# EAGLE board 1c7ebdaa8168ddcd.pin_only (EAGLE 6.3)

Size 35.57 x 21.59 mm. Coordinates in mm from the lower left corner, seen from the top.
Outline: 0,19.05 0,2.54 arc90 2.54,0 33.02,0 arc90 35.56,2.54 35.56,19.05 arc90 33.4,21.59 2.54,21.59 arc90 0,19.05
Copper layers (1*16): Top 0.035mm / dielectric 1.5mm / Bottom 0.035mm
Design rules "adafruit *": minimum track width 8mil, minimum drill 15.5mil, track to track 8mil, track to pad 8mil, pad to pad 8mil, via to via 8mil, smd to smd 8mil, copper to edge 10mil, drill to drill 8mil, minimum pad ring 10mil, minimum via ring 8mil, stop-mask expansion 2mil, vias tented up to drill 20mil, thermal gap 10mil

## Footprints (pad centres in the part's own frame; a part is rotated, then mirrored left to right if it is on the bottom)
JSTPH2 = smd 1 x 4.6: 1 -1,-3.7; 2 1,-3.7 | smd 1.6 x 3.4: NC1 -3.4,1.5; NC2 3.4,1.5
0805-NO = smd 1.3 x 1.5: 1 -0.95,0; 2 0.95,0
EIA3528-21/B-R = smd 1.95 x 2.5: + 1.525,0; - -1.525,0
USB_HOST-PTH = drill 0.95 long: D+ 1,6.52; D- -1,6.52; GND 3.5,6.52; VBUS -3.5,6.52 | drill 2.3 pad 2.9: S1 -6.57,3.81; S2 6.57,3.81
FIDUCIAL_1MM = smd 1 x 1: 1 0,0
1X06-CLEANBIG = drill 1.016 pad 1.778 octagon: 1 -6.35,0; 2 -3.81,0; 3 -1.27,0; 4 1.27,0; 5 3.81,0; 6 6.35,0
1X02_ROUND = drill 1 pad 1.778: 1 -1.27,0; 2 1.27,0
INDUCTOR_5X5MM_TDK_VLC5045 = smd 2 x 5: P$1 -1.6,0; P$2 1.6,0
CHIPLED_0805_NOOUTLINE = smd 1.2 x 1.2: A 0,-1.05; C 0,1.05
SC59-BEC = smd 1 x 1.4: B -0.95,-1.2; C 0,1.2; E 0.95,-1.2
PVQFN-16 = smd 1.05 x 0.35: 1 -2.1,0.975; 2 -2.1,0.325; 3 -2.1,-0.325; 4 -2.1,-0.975; 9 2.1,-0.975; 10 2.1,-0.325; 11 2.1,0.325; 12 2.1,0.975 | smd 0.35 x 1.05: 5 -0.975,-2.1; 6 -0.325,-2.1; 7 0.325,-2.1; 8 0.975,-2.1; 13 0.975,2.1; 14 0.325,2.1; 15 -0.325,2.1; 16 -0.975,2.1 | drill 0.4: P$18 0,0; P$19 -0.9,0.9; P$20 0.9,0.9; P$21 0.9,-0.9; P$22 -0.9,-0.9 | smd 2.7 x 2.7: THERMAL 0,0
SOT23-5 = smd 0.55 x 1.2: 1 -0.95,-1.3; 2 0,-1.3; 3 0.95,-1.3; 4 0.95,1.3; 5 -0.95,1.3
MOUNTINGHOLE_2.5_PLATED = drill 2.5 pad 3.2: P$1 0,0
TERMBLOCK_1X2-3.5MM = drill 1 pad 2.184: 1 1.8,0; 2 -1.7,0
4UCONN_20329 = smd 1 x 2: BASE@1 -0.75,-2; BASE@2 0.75,-2 | smd 0.4 x 1.35: D+ 0,0.775; D- -0.65,0.775; GND 1.3,0.775; ID 0.65,0.775; VBUS -1.3,0.775 | drill 0.7 offset: SPRT@1 -3.3,0.9; SPRT@2 3.3,0.9 | drill 0.6 pad 2.5 square: SPRT@3 -3.6,-1.9; SPRT@4 3.6,-1.9 | hole 0.7: -1.95,0; 1.95,0

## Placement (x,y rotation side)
B1  1.8-5V  [JSTPH2]  11.94,3.56 180 top
C1  10uF  [0805-NO]  18.29,13.08 270 top
C2  2.2uF  [0805-NO]  28.19,4.95 270 top
C4  0.1uF  [0805-NO]  20.07,13.08 270 top
C5  100uF/6V  [EIA3528-21/B-R]  25.78,2.79 90 top
C6  10µF  [0805-NO]  6.86,10.92 270 top
CN1  USBA_FEMALE  [USB_HOST-PTH]  37.08,10.79 90 top
FID2  FIDUCIAL""  [FIDUCIAL_1MM]  10.69,3.15 0 top
FID3  FIDUCIAL""  [FIDUCIAL_1MM]  33.78,20.19 0 top
JP1  [1X06-CLEANBIG]  21.59,20.32 0 top
JP2  [1X02_ROUND]  11.43,20.32 0 top
L1  VLC5045-6.8uH  [INDUCTOR_5X5MM_TDK_VLC5045]  24.02,14.13 0 top
LBO  RED  [CHIPLED_0805_NOOUTLINE]  6.73,2.16 180 top
LED3  ORANGE  [CHIPLED_0805_NOOUTLINE]  8.38,19.56 180 top
LED4  GREEN  [CHIPLED_0805_NOOUTLINE]  5.46,19.56 0 top
PWR  BLUE  [CHIPLED_0805_NOOUTLINE]  32.57,1.36 90 top
Q1  MMUN2133LT1G  [SC59-BEC]  9.91,11.81 0 top
R1  1.87Mohm  [0805-NO]  18.29,6.86 180 top
R2  340K  [0805-NO]  19.18,9.65 270 top
R3  1.87Mohm  [0805-NO]  22.99,3.05 270 top
R4  200K  [0805-NO]  21.08,3.05 270 top
R5  1K  [0805-NO]  29.08,1.27 180 top
R6  470  [0805-NO]  8.76,15.75 270 top
R7  1K  [0805-NO]  6.86,15.75 270 top
R8  2k  [0805-NO]  11.56,14.86 90 top
R9  75K 1%  [0805-NO]  27.99,8.64 270 top
R10  49.9K 1%  [0805-NO]  27.97,12.25 90 top
R11  75K 1%  [0805-NO]  30.99,20.19 180 top
R12  49.9K 1%  [0805-NO]  27.94,15.88 270 top
R13  340K  [0805-NO]  18.64,3.17 90 top
R20  1K  [0805-NO]  6.86,6.73 90 top
U1  TPS61090RSAR  [PVQFN-16]  23.76,8.43 180 top
U2  MCP73831T-2ACI/OT  [SOT23-5]  14.61,14.86 90 top
U$10  MOUNTINGHOLE2.5  [MOUNTINGHOLE_2.5_PLATED]  2.54,19.05 0 top
U$12  MOUNTINGHOLE2.5  [MOUNTINGHOLE_2.5_PLATED]  2.54,2.54 0 top
U$13  [SYMBOL_PLUS]  9.4,8.89 0 top
U$25  [SYMBOL_PLUS]  34.67,6.35 0 top
U$26  [SYMBOL_MINUS]  34.67,15.24 0 top
U$28  [ADAFRUIT_2.5MM]  17.14,15.11 0 top
U$29  [ADAFRUIT_5MM]  4.45,0.38 90 bottom
X1  [TERMBLOCK_1X2-3.5MM]  33.4,10.67 90 top
X2  microUSB  [4UCONN_20329]  4.32,10.79 270 top

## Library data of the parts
B1 C1 C2 C4-C6 CN1 JP2 L1 LBO LED3 LED4 PWR R1-R13 R20 U1 U2 U$13 U$25 U$26 U$28 U$29 X1 X2 = microbuilder
FID2 U$10 U$12 = microbuilder; BOM: EXCLUDE
FID3 = microbuilder; BOM: EXCLUDE; COMPANY: ADAFRUIT INDUSTRIES; DRAWN: KTOWN; REV: A
JP1 = adafruit
Q1 = transistor

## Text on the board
tPlace: Chrg | USB | GND | Bat | EN | GND | LB | GND | 5V | Power | Boost | 500C | PWR | Low | adafruit
bPlace: USB | GND | Bat | EN | GND | LBO | GND | 5Vo | PowerBoost 500 Charger | TPS61090 DC Boost | 500-1000mA from 3.7V LiPo | 5.2V output | 500mA Charge Current | 3.2V Low Batt Detect | Apple Charge Resistors

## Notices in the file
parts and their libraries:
microbuilder: This work is placed in the public domain, and may be freely used for commercial and non-commercial work with the following conditions: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
